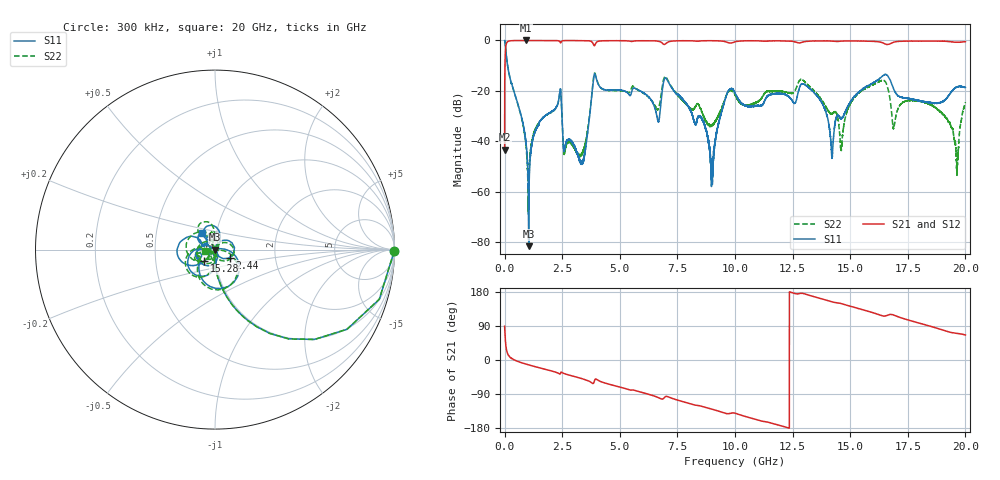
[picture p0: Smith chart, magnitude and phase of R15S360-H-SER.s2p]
!{R15S360}
!Johanson Technology Inc.
!www.johansontechnology.com
!Test Board Conditions:
!Substrate Type  RO4350B
!Substrate Thickness  20 mil
!Substrate Dk  3.66
!TL Type: GCPW
!TL Trace Width  34 mil
!TL Gap  10 mil
!Electrode orientation  Horizontal
!DUT TOPOLOGY	SERIES
!Mounting Pad LxW  26x52 mil
! Created Sat Feb  6 14:26:56 2021
# hz S ma R 50
! 2 Port Network Data from SP1.SP block
! freq  magS11  angS11  magS21  angS21  magS12  angS12  magS22  angS22
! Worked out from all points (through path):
!   20001 points, 300 kHz to 20 GHz, reference 50 ohm
!   highest |S21| = 0.00 dB at 919.3 MHz (marker M1); lowest = -43.4 dB at 300 kHz (marker M2)
!   group delay of S21, straight-line fit = 41.2 ps
!   lowest |S11| = -81.7 dB at 1.047 GHz (marker M3), VSWR 1.00, Z = 50 - j0.00808 ohm
!   |S11| at or under -10 dB: 130.8 MHz to end of sweep
!   |S22| runs from -69.0 to 0.0 dB; largest |S21 - S12| = 0.014
!   S11 on the Smith chart (normalised r, x): 300 kHz: open; 2.44 GHz: 1.18, -0.11; 15.28 GHz: 0.88, -0.11; 20 GHz: 0.85, +0.16
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300000  0.9979 -0.6  0.006794 89.0  0.00683 89.2  0.9983 -0.5
1.283e8  0.3215 -72.6  0.9454 17.1  0.945 17.1  0.3226 -72.7
9.193e8  0.01008 -99.6  0.9998 -10.6  0.9991 -10.6  0.009433 -102.1
1.0473e9  8.259e-05 -101.8  0.9993 -12.8  0.9989 -12.9  0.001442 94.9
2.4403e9  0.09503 -27.9  0.9026 -33.0  0.9038 -33.0  0.0941 -42.2
2.6193e9  0.008025 30.9  0.9945 -36.5  0.9949 -36.5  0.006444 12.5
3.3343e9  0.003917 35.2  0.9953 -48.8  0.9947 -48.8  0.005622 -25.4
3.9293e9  0.2139 -91.5  0.8283 -50.8  0.8284 -50.8  0.2191 -97.0
6.6673e9  0.02451 -142.0  0.9681 -99.1  0.968 -99.1  0.0433 -125.0
7.0343e9  0.1706 -152.6  0.8943 -96.0  0.8948 -96.0  0.1792 -156.9
8.5813e9  0.02727 155.4  0.9825 -122.7  0.9837 -122.6  0.03613 -177.2
9.0033e9  0.002103 42.0  0.9866 -129.9  0.9875 -129.9  0.0211 -122.3
1.00003e10  0.09131 177.1  0.9398 -140.4  0.9398 -140.4  0.08348 156.8
1.33343e10  0.102 76.0  0.9739 168.8  0.9727 168.7  0.1102 93.3
1.42083e10  0.004864 -34.0  0.969 153.6  0.9706 153.5  0.03516 124.4
1.46233e10  0.02854 -159.8  0.9709 148.5  0.9743 148.6  0.008 -170.2
1.52773e10  0.08703 -132.5  0.975 137.2  0.9776 137.2  0.08191 -135.5
1.66673e10  0.1864 162.6  0.8406 119.1  0.831 119.5  0.09793 111.3
1.68993e10  0.1054 146.9  0.9256 118.2  0.9225 118.7  0.01869 -36.2
1.89083e10  0.05796 146.4  0.9697 81.3  0.9691 81.4  0.03788 -149.8
1.96193e10  0.1192 142.9  0.921 70.2  0.9202 70.6  0.002977 0.8
2e10  0.1165 127.8  0.9441 65.9  0.942 65.7  0.05776 -172.9
